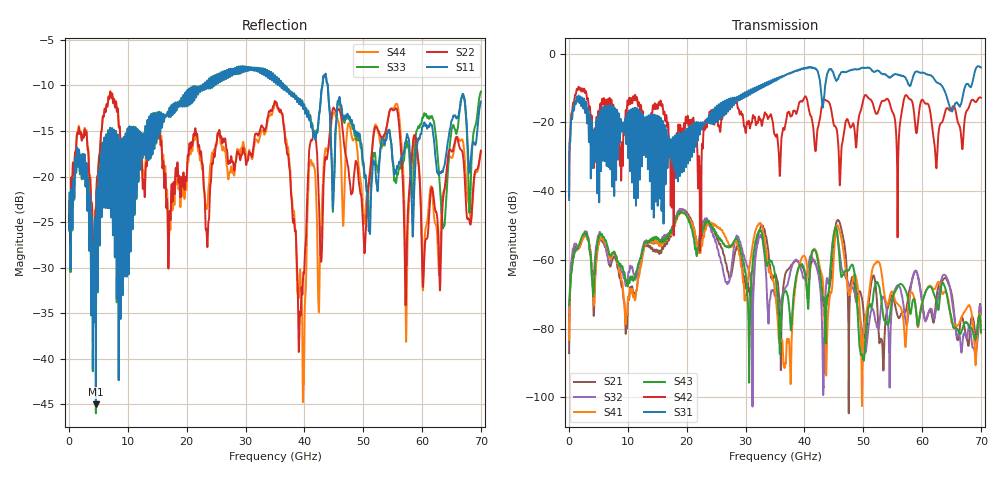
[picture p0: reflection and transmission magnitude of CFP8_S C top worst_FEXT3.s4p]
! AWR Design Environment (8415) Tue Jan 08 14:28:58 2019
! Document = 'CFP8 Channel_S_2'
! nPorts: 4, nXvals: 7001
# HZ S DB R 50
!Freq DBS11 AngS11 DBS12 AngS12 DBS13 AngS13 DBS14 AngS14
!	DBS21 AngS21 DBS22 AngS22 DBS23 AngS23 DBS24 AngS24
!	DBS31 AngS31 DBS32 AngS32 DBS33 AngS33 DBS34 AngS34
!	DBS41 AngS41 DBS42 AngS42 DBS43 AngS43 DBS44 AngS44
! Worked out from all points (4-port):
!   7000 points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, 10 MHz to 70 GHz, reference 50 ohm
!   strongest paths, dB at 10 MHz, 17.51 GHz, 35.01 GHz, 52.51 GHz, 70 GHz:
!     S31: -42.6, -30.3, -7.5, -5.0, -4.0
!     S42: -41.5, -36.6, -23.7, -17.0, -12.8
!     S43: -73.2, -50.7, -64.4, -66.9, -81.1
!     S41: -83.3, -51.3, -69.3, -60.5, -81.3
!     S32: -77.5, -50.3, -70.5, -79.6, -75.8
!     S21: -87.1, -51.6, -64.8, -77.8, -75.1
!   lowest |S11| = -45.0 dB at 4.56 GHz (marker M1), VSWR 1.01, Z = 49.8 + j0.54 ohm
!   |S11| at or under -10 dB: start of sweep to 22.76 GHz; 36.66 GHz to 43.06 GHz (6.402 GHz wide, 16.1 % of centre); 43.97 GHz to end of sweep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
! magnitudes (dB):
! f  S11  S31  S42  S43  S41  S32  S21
! 10 MHz  -25.9  -42.6  -41.5  -73.2  -83.3  -77.5  -87.1
! 4.56 GHz  -45.0  -23.8  -23.2  -58.3  -61.7  -56.5  -61.1
! 32.45 GHz  -8.6  -10.1  -19.3  -51.4  -49.5  -53.2  -51.2
! 43.73 GHz  -9.3  -7.3  -13.7  -73.8  -92.5  -66.3  -73.1
! 45.68 GHz  -11.7  -7.6  -24.8  -53.8  -50.0  -53.7  -48.4
! 50.4 GHz  -19.9  -4.1  -12.0  -82.6  -76.8  -86.9  -86.5
! 70 GHz  -11.8  -4.0  -12.8  -81.1  -81.3  -75.8  -75.1
